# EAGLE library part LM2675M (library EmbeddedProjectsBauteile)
1A-Spannungsregler
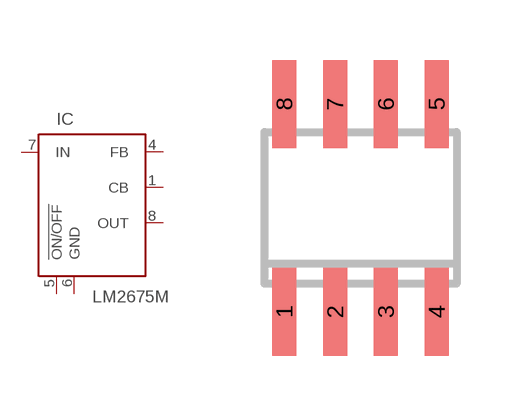
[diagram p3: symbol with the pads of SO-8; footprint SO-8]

Designator prefix IC

## LM2675M (EP: 400974)  [SO-8]
1  CB  in
4  FB  in
5  !ON/OFF  in
6  GND  pwr
7  IN  in
8  OUT  pas

## Footprint SO-8 (pad centres in mm)
smd 0.6 x 2.2: 1 -1.905,-2.6; 2 -0.635,-2.6; 3 0.635,-2.6; 4 1.905,-2.6; 5 1.905,2.6; 6 0.635,2.6; 7 -0.635,2.6; 8 -1.905,2.6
